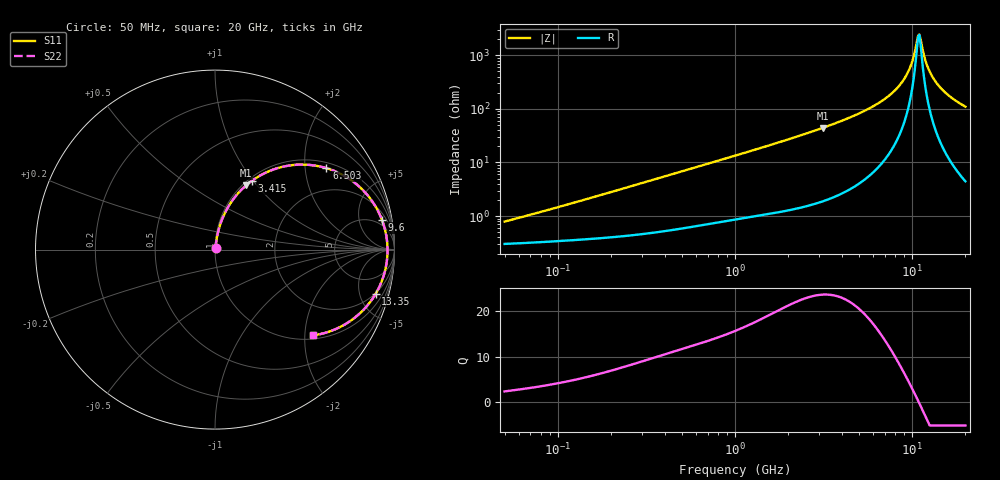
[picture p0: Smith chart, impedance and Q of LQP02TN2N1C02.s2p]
!Murata Part Number: LQP02TN2N1C02
!These Parameters are Measured in Series Mode Connection
!  o--[Z]--o
!Port1  Port2
!  o-------o
!Freq. Start=50[MHz] Stop=20[GHz], 401[Steps]
# Hz S RI R 50
!Freq.(Hz) S11(Real) S11(Imag) S21(Real) S21(Imag) S12(Real) S12(Imag) S22(Real) S22(Imag)
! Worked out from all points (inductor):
!   401 points, 50 MHz to 20 GHz, reference 50 ohm
!   read as one part in series: L = 2.28 nH near 65.47 MHz
!   highest Q = 23.5 at 3.122 GHz (marker M1), where L = 2.25 nH
!   self-resonance near 10.82 GHz
!   S11 on the Smith chart (normalised r, x): 50 MHz: 1.01, +0.01; 3.415 GHz: 1.04, +0.98; 6.503 GHz: 1.17, +2.59; 9.6 GHz: 3, +10; 13.35 GHz: 1.94, -6.91; 20 GHz: 1.09, -2.20
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5e7  0.00307 0.00725  0.9969 -0.00725  0.9969 -0.00725  0.00307 0.00725
1.364002e8  0.00399 0.0191  0.996 -0.0191  0.996 -0.0191  0.00399 0.0191
3.721004e8  0.00758 0.0503  0.9924 -0.0503  0.9924 -0.0503  0.00758 0.0503
1e9  0.0256 0.1291  0.9744 -0.1291  0.9744 -0.1291  0.0256 0.1291
1.793498e9  0.0647 0.2224  0.9353 -0.2224  0.9353 -0.2224  0.0647 0.2224
2.728004e9  0.1354 0.3212  0.8646 -0.3212  0.8646 -0.3212  0.1354 0.3212
3.121702e9  0.1731 0.3576  0.8269 -0.3576  0.8269 -0.3576  0.1731 0.3576
3.415248e9  0.204 0.3822  0.796 -0.3822  0.796 -0.3822  0.204 0.3822
4.748272e9  0.3703 0.4598  0.6297 -0.4598  0.6297 -0.4598  0.3703 0.4598
6.503449e9  0.6205 0.4539  0.3795 -0.4539  0.3795 -0.4539  0.6205 0.4539
7.442007e9  0.7444 0.3966  0.2556 -0.3966  0.2556 -0.3966  0.7444 0.3966
8.644534e9  0.8686 0.2792  0.1314 -0.2792  0.1314 -0.2792  0.8686 0.2792
9.600142e9  0.9306 0.1648  0.0694 -0.1648  0.0694 -0.1648  0.9306 0.1648
1.004137e10  0.9476 0.1097  0.0524 -0.1097  0.0524 -0.1097  0.9476 0.1097
1.066139e10  0.9598 0.0329  0.0402 -0.0329  0.0402 -0.0329  0.9598 0.0329
1.098561e10  0.9612 -0.00617  0.0388 0.00617  0.0388 0.00617  0.9612 -0.00617
1.115139e10  0.9607 -0.0257  0.0393 0.0257  0.0393 0.0257  0.9607 -0.0257
1.183995e10  0.9508 -0.1031  0.0492 0.1031  0.0492 0.1031  0.9508 -0.1031
1.220001e10  0.9412 -0.1407  0.0588 0.1407  0.0588 0.1407  0.9412 -0.1407
1.334722e10  0.8958 -0.245  0.1042 0.245  0.1042 0.245  0.8958 -0.245
1.573793e10  0.7662 -0.389  0.2338 0.389  0.2338 0.389  0.7662 -0.389
2e10  0.5462 -0.4781  0.4538 0.4781  0.4538 0.4781  0.5462 -0.4781
